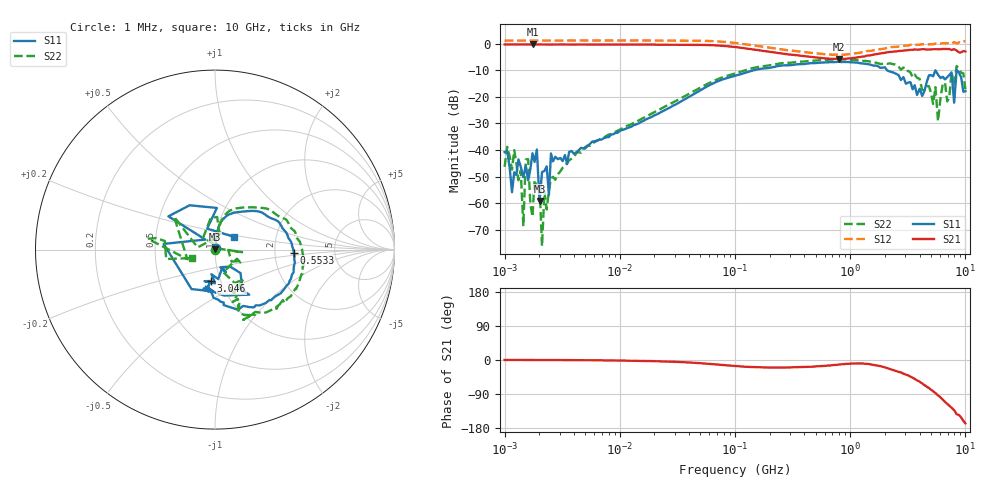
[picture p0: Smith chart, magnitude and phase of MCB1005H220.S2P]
!Agilent Technologies,E5071C,MY46111244,A.11.31
!Date: Tue May 07 16:29:17 2019
!Data & Calibration Information:
!Freq	S11:SOLT2(ON)	S21:SOLT2(ON)	S12:SOLT2(ON)	S22:SOLT2(ON)
# Hz S dB R 50
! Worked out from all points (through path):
!   201 points, 1 MHz to 10 GHz, reference 50 ohm
!   highest |S21| = -0.29 dB at 1.746 MHz (marker M1); lowest = -5.8 dB at 798.8 MHz (marker M2)
!   group delay of S21, straight-line fit = 42 ps
!   lowest |S11| = -59.3 dB at 2.009 MHz (marker M3), VSWR 1.00, Z = 49.9 + j0.0928 ohm
!   |S11| at or under -10 dB: start of sweep to 145.6 MHz; 2.092 GHz to 8.388 GHz (6.296 GHz wide, 120 % of centre); 8.422 GHz to end of sweep
!   |S22| runs from -76.2 to -5.9 dB; largest |S21 - S12| = 0.51
!   S11 on the Smith chart (normalised r, x): 1 MHz: 1.01, +0.01; 553.3 MHz: 2.56, -0.11; 3.046 GHz: 0.90, -0.33; 10 GHz: 1.22, +0.18
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1000000  -40.81 53.9  -0.30 0.0  1.13 -0.8  -46.34 -67.0
1159128  -55.90 129.1  -0.30 0.1  1.17 -0.8  -47.40 -85.8
1380384  -46.27 67.7  -0.31 0.0  1.14 -0.8  -47.79 -60.3
1453604  -50.23 40.6  -0.31 -0.0  1.14 -0.8  -68.68 64.6
1526823  -46.03 57.5  -0.29 -0.0  1.14 -0.8  -43.60 -67.0
1600043  -51.42 169.8  -0.33 0.0  1.11 -0.5  -43.42 -42.3
1746481  -41.22 32.7  -0.29 -0.0  1.15 -1.1  -65.14 -40.9
1905461  -39.86 123.9  -0.30 0.1  1.12 -0.8  -54.03 48.8
2009005  -59.25 121.5  -0.32 -0.1  1.16 -1.0  -52.70 -16.8
2112549  -48.33 -109.9  -0.30 -0.1  1.15 -1.0  -76.21 -29.8
2216092  -47.91 86.4  -0.30 -0.1  1.17 -1.1  -55.77 -0.5
4810209  -39.42 87.9  -0.32 -0.5  1.18 -1.3  -39.77 78.5
2.206931e7  -26.12 84.6  -0.37 -3.5  1.18 -3.7  -24.81 83.6
1.047129e8  -11.86 55.6  -1.36 -16.4  0.18 -16.3  -10.95 55.9
4.810209e8  -7.34 3.0  -5.15 -17.5  -3.58 -16.3  -6.41 2.4
5.533258e8  -7.14 -2.2  -5.35 -16.4  -3.78 -14.9  -6.21 -2.6
7.988146e8  -6.82 -16.1  -5.77 -12.0  -4.21 -9.7  -6.00 -15.8
2.206931e9  -10.48 -80.6  -3.11 -23.7  -1.30 -17.9  -7.40 -58.6
3.046413e9  -15.08 -97.1  -2.50 -38.5  -0.66 -31.0  -10.36 -65.1
5.786901e9  -11.68 -79.0  -2.14 -93.5  -0.08 -79.1  -29.15 5.3
8.390517e9  -9.92 144.5  -2.56 -142.9  0.06 -124.1  -8.41 170.8
1e10  -17.91 34.1  -2.95 -167.2  0.94 -146.9  -17.19 -160.0
